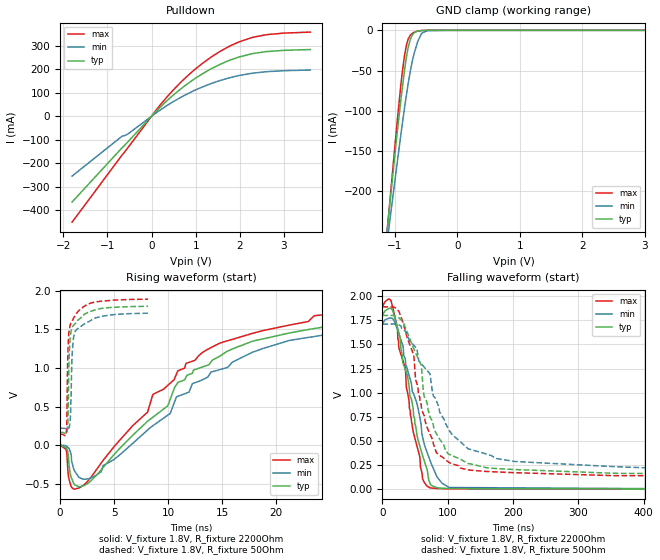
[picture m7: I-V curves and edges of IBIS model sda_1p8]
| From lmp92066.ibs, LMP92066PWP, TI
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|   sda_1p8 Model
[Model]   sda_1p8
Model_type   I/O_open_drain
Polarity   Non-Inverting
Vinl = 0.54
Vinh = 1.26
Vmeas = 0.9
Vref = 1.8
Cref = 100pF
Rref = 2200
|   typ   min   max
|   (nom PVT)   (fast PVT)   (slow PVT)
C_comp   2.070e-12   1.832e-12   2.430e-12
[Model spec]
|subparameter
Vinl   0.54   0.513   0.567
Vinh   1.26   1.197   1.323
| Where nom  PVT is Nominal Process, 1.8V, 25C
|   Fast PVT is Strong Process,  1.89V, -25C
|   Slow PVT is Weak Process,   1.71V, 125C
[Voltage Range]   1.8   1.71   1.89
|Junction Temperature
[Temperature Range]   25   125   -25
[Pullup Reference]   1.8   1.71   1.89
[Pulldown Reference]   0   0   0
[Power Clamp Reference]   1.8   1.71   1.89
[GND Clamp Reference]   0   0   0
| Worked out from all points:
|   slope of the pulldown table from 0 to 0.27 V, typ, clamps not added: 5.21 ohm
|   GND clamp passes 1 mA (typ) near -0.64 V on its own axis
|   falling waveform, V_fixture 1.8V, R_fixture 2200Ohm: 20-80 % time 32.3ns typ, 36.5ns min, 30.8ns max; typ from 1.8 V to 0.004 V
|   rising waveform, V_fixture 1.8V, R_fixture 2200Ohm: 20-80 % time 12.3ns typ, 12.3ns min, 12.1ns max; typ from 0.004 V to 1.8 V
|   falling waveform, V_fixture 1.8V, R_fixture 50Ohm: 20-80 % time 43.8ns typ, 61.1ns min, 38ns max; typ from 1.8 V to 0.166 V
|   rising waveform, V_fixture 1.8V, R_fixture 50Ohm: 20-80 % time 261ps typ, 276ps min, 267ps max; typ from 0.166 V to 1.8 V
[Pulldown]
|   Voltage   I(typ)   I(min)   I(max)
-1.8V     -365.5mA   -254.7mA   -451.4mA
-662.2mV  -133.1mA   -84.15mA   -163.9mA
-546.6mV  -111.2mA   -76.98mA   -136.9mA
226.1mV   44.24mA    30.64mA    54.83mA
682.9mV   119.8mA    82.88mA    148.7mA
1.114V    176.6mA    122mA      219.9mA
1.418V    209mA      144.1mA    260.8mA
1.704V    233.9mA    161mA      292.7mA
1.982V    252.8mA    173.8mA    317.3mA
2.275V    266.9mA    183.6mA    335.9mA
2.612V    276.2mA    190.4mA    348.2mA
3.6V      284.7mA    197.5mA    359.1mA
[GND Clamp]
|   Voltage   I(typ)   I(min)   I(max)
-1.8V     -761.7mA   -651mA     -804.9mA
-1.186V   -295.7mA   -299.9mA   -300.9mA
-997.2mV  -151.4mA   -184.9mA   -140.7mA
-905.4mV  -86.7mA    -129.7mA   -68.19mA
-847.4mV  -50.17mA   -96.83mA   -31.77mA
-817.2mV  -33.79mA   -80.76mA   -19.04mA
-783mV    -19.59mA   -63.84mA   -10.16mA
-712.8mV  -4.811mA   -35.16mA   -3.297mA
-635.5mV  -979.4uA   -13.95mA   -936.8uA
-575.3mV  -265.5uA   -4.168mA   -244.7uA
-476.5mV  -22.5uA    -354.2uA   -15.18uA
3.6V      0A         0A         0A
[POWER Clamp]
|   Voltage   I(typ)   I(min)   I(max)
-1.8V     0A         0A         0A
0V        0A         0A         0A
3.6V      0A         0A         0A
[Ramp]
R_load = 2200
|   typ   min   max
dV/dt_r   1.0776/1.22591e-08   1.02301/1.22472e-08   1.13197/1.20512e-08
dV/dt_f   1.0776/3.21976e-08   1.02301/3.65157e-08   1.13197/3.07804e-08
[Falling Waveform]
V_fixture = 1.8V
V_fixture_min = 1.71V
V_fixture_max = 1.89V
R_fixture = 2200Ohm
|   Time   V(typ)   V(min)   V(max)
0s        1.8V       1.71V      1.89V
10.89ns   1.874V     1.773V     1.969V
19.06ns   1.776V     1.725V     1.784V
35.1ns    1.239V     1.338V     1.255V
42.91ns   955.7mV    1.129V     764.2mV
52.84ns   566.7mV    888.9mV    448.5mV
61.38ns   353.3mV    542.6mV    110.1mV
70.82ns   96.79mV    336.9mV    24.7mV
102ns     10.06mV    20.56mV    6.571mV
527.5ns   3.995mV    5.477mV    3.388mV
[Rising Waveform]
V_fixture = 1.8V
V_fixture_min = 1.71V
V_fixture_max = 1.89V
R_fixture = 2200Ohm
|   Time   V(typ)   V(min)   V(max)
0s        3.995mV    5.477mV    3.388mV
548.4ps   -26.78mV   -4.982mV   -50.22mV
994.6ps   -400.9mV   -108.8mV   -524.5mV
1.741ns   -535.3mV   -412.8mV   -550.2mV
3.808ns   -313.6mV   -339.7mV   -225.8mV
11.66ns   881.1mV    673.2mV    1.059V
17.81ns   1.345V     1.203V     1.447V
23.53ns   1.509V     1.406V     1.675V
31.36ns   1.7V       1.543V     1.775V
65.75ns   1.8V       1.71V      1.89V
[Falling Waveform]
V_fixture = 1.8V
V_fixture_min = 1.71V
V_fixture_max = 1.89V
R_fixture = 50Ohm
|   Time   V(typ)   V(min)   V(max)
0s        1.8V       1.71V      1.89V
31.37ns   1.736V     1.656V     1.73V
48.02ns   1.453V     1.49V      1.388V
50.72ns   1.414V     1.47V      1.136V
59.59ns   1.284V     1.299V     854.1mV
62.53ns   1.019V     1.276V     783.4mV
67.28ns   918.2mV    1.239V     659.6mV
101.2ns   366.8mV    623.6mV    282.7mV
173.4ns   216.7mV    321.3mV    181.8mV
419.9ns   166mV      221.6mV    142.5mV
[Rising Waveform]
V_fixture = 1.8V
V_fixture_min = 1.71V
V_fixture_max = 1.89V
R_fixture = 50Ohm
|   Time   V(typ)   V(min)   V(max)
0s        166mV      221.1mV    142.5mV
577.5ps   155.4mV    213.7mV    168.1mV
613.7ps   160.9mV    213.2mV    263.3mV
729.4ps   352.9mV    216.6mV    1.244V
825.7ps   1.108V     231.9mV    1.472V
914.5ps   1.365V     292mV      1.545V
1.11ns    1.521V     1.18V      1.608V
1.275ns   1.556V     1.416V     1.653V
3.294ns   1.753V     1.648V     1.852V
8.146ns   1.797V     1.707V     1.889V
